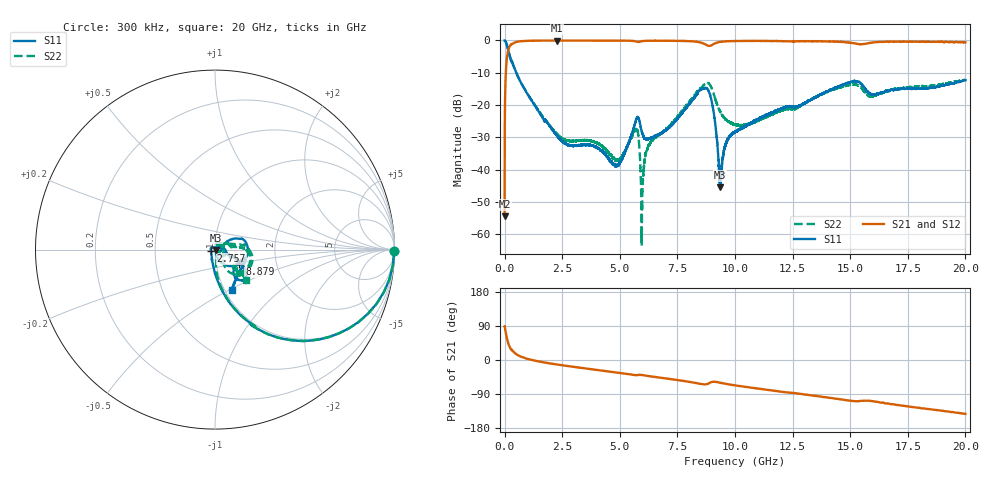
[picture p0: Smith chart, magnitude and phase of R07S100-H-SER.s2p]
!{R07S100}
!Johanson Technology Inc.
!www.johansontechnology.com
!Test Board Conditions:
!Substrate Type  RO4350B
!Substrate Thickness  10 mil
!Substrate Dk  3.66
!TL Type: GCPW
!TL Trace Width  21 mil
!TL Gap  20 mil
!Electrode orientation  Horizontal
!DUT TOPOLOGY	SERIES
!Mounting Pad LxW  16x21 mil
! Created Sat Feb  6 11:42:36 2021
# hz S ma R 50
! 2 Port Network Data from SP1.SP block
! freq  magS11  angS11  magS21  angS21  magS12  angS12  magS22  angS22
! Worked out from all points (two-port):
!   20001 points, 300 kHz to 20 GHz, reference 50 ohm
!   highest |S21| = -0.03 dB at 2.278 GHz (marker M1); lowest = -54.5 dB at 300 kHz (marker M2)
!   |S21| within 3 dB of the highest: 158.2 MHz to end of sweep
!   lowest |S11| = -45.5 dB at 9.346 GHz (marker M3), VSWR 1.01, Z = 50.5 - j0.204 ohm
!   |S11| at or under -10 dB: 504.3 MHz to end of sweep
!   |S22| runs from -63.7 to 0.0 dB; largest |S21 - S12| = 0.013
!   S11 on the Smith chart (normalised r, x): 300 kHz: open; 2.757 GHz: 0.96, -0.02; 8.879 GHz: 1.29, -0.21; 20 GHz: 1.08, -0.51
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300000  0.9994 -0.4  0.001894 89.2  0.001919 90.4  0.9991 -0.4
1.053e8  0.8305 -34.3  0.5531 55.9  0.5541 55.8  0.8311 -34.3
2.273e8  0.5684 -57.0  0.8199 33.3  0.8183 33.4  0.5679 -57.1
7.043e8  0.2236 -81.0  0.9717 9.0  0.9712 9.0  0.2242 -79.9
2.2783e9  0.03314 -128.0  0.9971 -11.9  0.9961 -11.9  0.03526 -71.0
2.7573e9  0.02417 -160.8  0.9954 -16.1  0.9954 -16.1  0.02785 -48.9
3.3343e9  0.02403 168.1  0.9955 -20.8  0.9951 -20.8  0.02837 -31.8
4.8863e9  0.01196 80.3  0.9934 -33.0  0.9941 -33.0  0.01423 20.3
5.7053e9  0.05913 -2.7  0.9633 -40.2  0.9625 -40.1  0.04316 29.9
5.9803e9  0.036 -44.9  0.9773 -39.7  0.9782 -39.8  0.004572 137.1
6.1883e9  0.02919 -25.5  0.9884 -41.9  0.9883 -41.8  0.02047 102.9
6.6673e9  0.03527 -2.1  0.9903 -45.9  0.9905 -45.9  0.03409 78.7
8.4873e9  0.1699 18.1  0.932 -62.9  0.9329 -62.9  0.1781 5.7
8.8793e9  0.1581 -30.8  0.8239 -61.1  0.8235 -61.1  0.213 -35.3
9.0953e9  0.06827 -67.5  0.8878 -57.3  0.8873 -57.3  0.1406 -58.8
9.3463e9  0.005307 -22.3  0.9503 -59.9  0.9502 -60.0  0.08102 -54.9
9.6293e9  0.02617 48.9  0.9715 -63.3  0.9707 -63.2  0.0589 -35.9
1.00003e10  0.03802 33.0  0.98 -67.0  0.9799 -67.0  0.05037 -14.1
1.33343e10  0.1224 -22.7  0.9725 -93.4  0.9731 -93.5  0.1236 7.2
1.51373e10  0.2341 -41.9  0.9083 -108.0  0.9074 -108.1  0.2082 -23.2
1.66673e10  0.1643 -17.8  0.9492 -115.1  0.9547 -115.4  0.1687 -43.2
2e10  0.2426 -66.9  0.9392 -142.2  0.9381 -142.1  0.2446 -44.5
